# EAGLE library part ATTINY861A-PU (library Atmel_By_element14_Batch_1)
8-bit Microcontroller
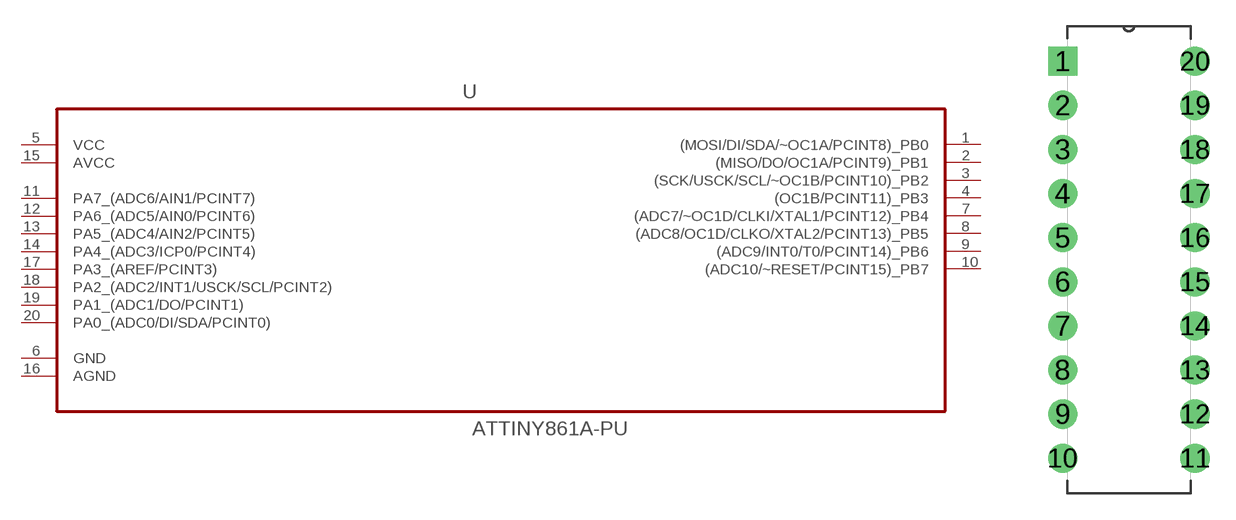
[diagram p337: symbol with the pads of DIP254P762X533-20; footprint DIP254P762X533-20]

Designator prefix U

## ATTINY861A-PU (DESCRIPTION: 8-bit Microcontroller; MPN: ATTINY861A-PU; OC_FARNELL: 1841627; OC_NEWARK: 12T1343; PACKAGE: DIP-20; SUPPLIER: Atmel)  [DIP254P762X533-20]
1  (MOSI/DI/SDA/~OC1A/PCINT8)_PB0
2  (MISO/DO/OC1A/PCINT9)_PB1
3  (SCK/USCK/SCL/~OC1B/PCINT10)_PB2
4  (OC1B/PCINT11)_PB3
5  VCC  pwr
6  GND  pas
7  (ADC7/~OC1D/CLKI/XTAL1/PCINT12)_PB4
8  (ADC8/OC1D/CLKO/XTAL2/PCINT13)_PB5
9  (ADC9/INT0/T0/PCINT14)_PB6
10  (ADC10/~RESET/PCINT15)_PB7
11  PA7_(ADC6/AIN1/PCINT7)
12  PA6_(ADC5/AIN0/PCINT6)
13  PA5_(ADC4/AIN2/PCINT5)
14  PA4_(ADC3/ICP0/PCINT4)
15  AVCC  pwr
16  AGND  pas
17  PA3_(AREF/PCINT3)
18  PA2_(ADC2/INT1/USCK/SCL/PCINT2)
19  PA1_(ADC1/DO/PCINT1)
20  PA0_(ADC0/DI/SDA/PCINT0)

## Footprint DIP254P762X533-20 (pad centres in mm)
drill 1.118 square: 1 -7.62,22.86
drill 1.118: 2 -7.62,20.32; 3 -7.62,17.78; 4 -7.62,15.24; 5 -7.62,12.7; 6 -7.62,10.16; 7 -7.62,7.62; 8 -7.62,5.08; 9 -7.62,2.54; 10 -7.62,0; 11 0,0; 12 0,2.54; 13 0,5.08; 14 0,7.62; 15 0,10.16; 16 0,12.7; 17 0,15.24; 18 0,17.78; 19 0,20.32; 20 0,22.86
